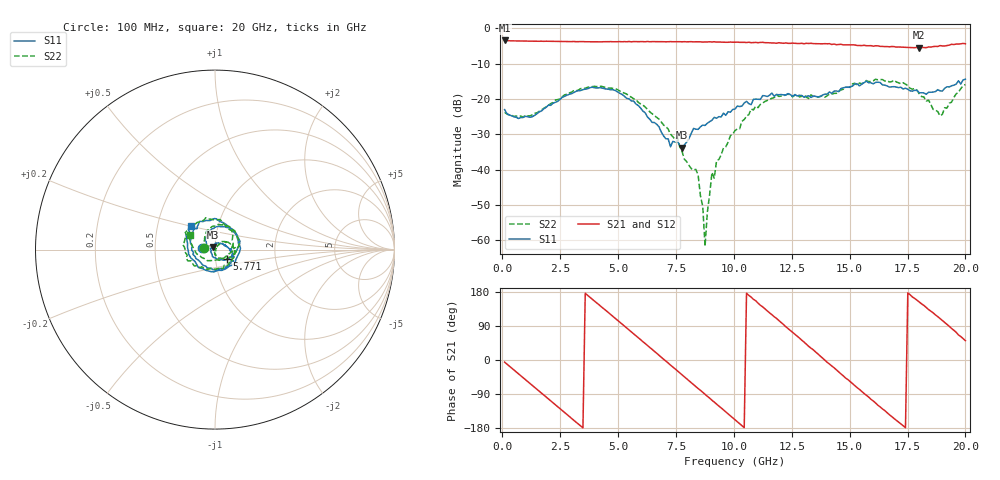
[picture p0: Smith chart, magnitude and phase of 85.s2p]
!Agilent Technologies,N5230C,MY49001569,A.09.33.09
!Agilent N5230C: A.09.33.09
!Date: Tuesday, July 28, 2015 10:12:01
!Correction: S11(Full 2 Port(1,2))
!S21(Full 2 Port(1,2))
!S12(Full 2 Port(1,2))
!S22(Full 2 Port(1,2))
!S2P File: Measurements: S11, S21, S12, S22:
# Hz S  dB  R 50
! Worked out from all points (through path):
!   201 points, 100 MHz to 20 GHz, reference 50 ohm
!   highest |S21| = -3.39 dB at 100 MHz (marker M1); lowest = -5.5 dB at 18.01 GHz (marker M2)
!   group delay of S21, straight-line fit = 143 ps
!   lowest |S11| = -33.8 dB at 7.761 GHz (marker M3), VSWR 1.04, Z = 48.6 + j1.5 ohm
!   |S11| at or under -10 dB: start of sweep to end of sweep
!   |S22| runs from -61.7 to -14.4 dB; largest |S21 - S12| = 0.019
!   S11 on the Smith chart (normalised r, x): 100 MHz: 0.87, +0.02; 5.771 GHz: 1.13, -0.12; 20 GHz: 0.74, +0.20
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1e8  -23.00 171.2  -3.39 -5.7  -3.42 -5.8  -23.78 170.0
9.955e8  -24.90 151.2  -3.57 -51.7  -3.56 -51.9  -24.67 155.9
1.7915e9  -22.77 135.1  -3.64 -92.7  -3.63 -92.7  -22.67 142.6
3.483e9  -17.35 70.7  -3.72 -179.0  -3.76 -179.4  -17.00 80.0
4.677e9  -17.41 15.1  -3.73 120.1  -3.76 120.3  -16.91 26.2
5.7715e9  -21.42 -39.5  -3.73 64.0  -3.75 63.8  -20.13 -23.3
6.7665e9  -27.86 -111.0  -3.74 12.5  -3.69 12.5  -25.71 -65.1
7.7615e9  -33.76 131.3  -3.77 -38.7  -3.77 -39.2  -34.80 -94.6
8.458e9  -28.61 77.9  -3.77 -75.3  -3.81 -75.4  -41.57 -57.6
8.657e9  -27.39 62.7  -3.85 -85.3  -3.80 -85.8  -50.46 -39.6
8.7565e9  -27.50 56.2  -3.81 -90.4  -3.82 -90.9  -61.74 -125.7
9.055e9  -26.01 39.3  -3.82 -106.3  -3.85 -106.4  -40.83 39.4
1.005e10  -22.85 10.5  -3.90 -157.9  -3.96 -158.1  -28.96 55.4
1.09455e10  -20.02 -12.2  -3.94 156.3  -3.93 155.0  -22.04 27.5
1.19405e10  -18.80 -43.0  -4.04 104.3  -4.12 103.5  -19.26 -5.4
1.3433e10  -19.16 -127.4  -4.29 26.8  -4.28 26.1  -19.28 -72.0
1.4229e10  -18.41 -172.0  -4.54 -15.7  -4.29 -16.1  -18.64 -111.9
1.5224e10  -15.75 137.1  -4.67 -67.5  -4.71 -68.2  -15.53 -164.1
1.67165e10  -16.62 57.7  -5.19 -144.3  -5.16 -144.1  -15.15 118.0
1.801e10  -18.25 -48.7  -5.47 152.8  -5.56 152.3  -18.63 33.5
1.89055e10  -17.68 -143.5  -4.85 109.4  -5.13 108.9  -24.78 -79.8
2e10  -14.40 135.7  -4.33 51.1  -4.39 51.1  -15.92 150.5
